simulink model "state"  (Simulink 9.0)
settings: Solver=VariableStepAuto  StartTime=0.0  StopTime=dps_simdata.endTime  RelTol=1e-3
undefined symbols (not defined in the file or in its folder): a, b, dps_simdata, Q, R, SamplePeriod
libraries: dps x5

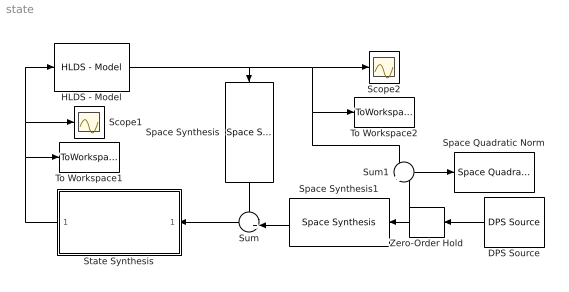
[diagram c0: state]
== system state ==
  DPS Source : dps/DPS Source  equation=dps_simdata.w  responseVar=0  showInput=off  pointsCoord=dps_simdata.points  elementsVar=[]  samplePeriod=dps_simdata.T
  HLDS - Model : dps/Controlled Systems/HLDS - Model  StepResponse=dps_simdata.H  samplePeriod=dps_simdata.T  u_step=1
  Scope1 : Scope
  Scope2 : Scope
  Space Quadratic Norm : dps/Quadratic norms/Space Quadratic Norm  StepResponse=dps_simdata.H  showNorm=on
  Space Synthesis : dps/Space Synthesis/Space Synthesis  PCH=dps_simdata.H  weights=dps_simdata.weights
  Space Synthesis1 : dps/Space Synthesis/Space Synthesis  PCH=dps_simdata.H  weights=dps_simdata.weights
  State Synthesis : Subsystem  AncestorBlock=dps/Temporal Synthesis/State Synthesis
  Sum : Sum  Inputs=-+|
  Sum1 : Sum  Inputs=-|+
  To Workspace1 : ToWorkspace  VariableName=simU  SaveFormat=Structure  SampleTime=-1
  To Workspace2 : ToWorkspace  VariableName=simY  SaveFormat=Structure  SampleTime=-1
  Zero-Order Hold : ZeroOrderHold  SampleTime=-1
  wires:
  HLDS - Model/1 -> Space Synthesis/1, To Workspace2/1, Sum1/1, Scope2/1
  State Synthesis/1(u) -> To Workspace1/1, HLDS - Model/1, Scope1/1
  DPS Source/1 -> Zero-Order Hold/1
  Zero-Order Hold/1 -> Sum1/2, Space Synthesis1/1
  Space Synthesis/1 -> Sum/1
  Space Synthesis1/1 -> Sum/2
  Sum/1 -> State Synthesis/1(y)
  Sum1/1 -> Space Quadratic Norm/1

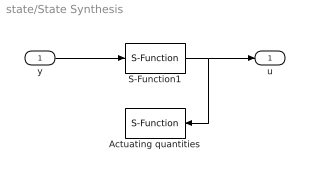
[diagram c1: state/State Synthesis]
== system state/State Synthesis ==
  y : Inport
  Actuating quantities : S-Function  FunctionName=sfun_scope  Parameters=length(dps_simdata.H)  SFunctionDeploymentMode=off  EnableBusSupport=off
  S-Function1 : S-Function  FunctionName=sfun_state  Parameters=a,b,SamplePeriod,Q,R  SFunctionDeploymentMode=off  EnableBusSupport=off
  u : Outport
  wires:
  S-Function1/1 -> u/1, Actuating quantities/1
  y/1 -> S-Function1/1
